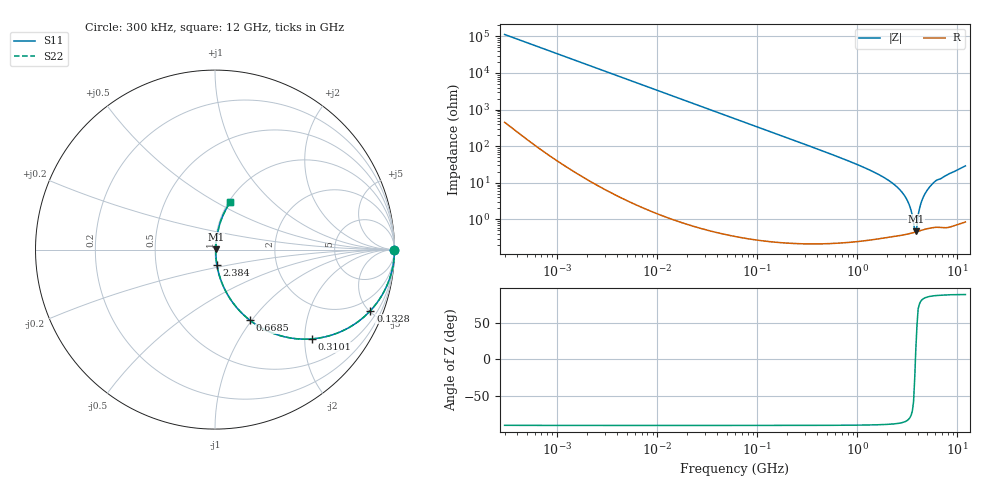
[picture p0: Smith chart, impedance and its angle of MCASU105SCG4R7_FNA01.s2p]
! MCASU105SCG4R7_FNA01  S-PARAMETER MODEL  ( Standard Model )
! Model Generated by TAIYO YUDEN Corporation (http://www.ty-top.com)
! Version 1.0
! TAIYO YUDEN Control No. 230609
! Copyright(c) 2023 TAIYO YUDEN CO.,LTD. All Rights Reserved.
! Product Description (link to TY-COMPAS)
! https://ds.yuden.co.jp/TYCOMPAS/or/detail?pn=MCASU105SCG4R7CFNA01&u=M
! Products Name : Multilayer Ceramic Capacitors
! Characteristics :
!  Capacitance : 4.7 [pF] , Rated Voltage : 50 [V] , TCC : CG / C0G
!  Case Size : 1.0 x 0.5 / 0.039 x 0.02 [mm/inch] , Thickness : 0.5 / 0.02 [mm/inch]
!  (Conditions: Temperature = 25 [degC] , DC Bias Voltage = 0 [V])
! External Node Assignments :
!  1  o---| |---o  2
! GND o---------o GND
! Frequency Range : 0.3MHz  -  12000MHz  [ 401 STEP ]
# MHZ S RI R 50
! Freq[MHz].  S11 Real  S11 Imag  S21 Real  S21 Imag  S12 Real  S12 Imag  S22 Real  S22 Imag
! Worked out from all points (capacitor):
!   401 points, 300 kHz to 12 GHz, reference 50 ohm
!   read as one part in series: C = 4.7 pF near 316.3 kHz
!   lowest |Z| = 471 mohm at 3.841 GHz (marker M1)
!   series resonance near 3.805 GHz, so ESL is about 370 pH
!   S11 on the Smith chart (normalised r, x): 300 kHz: open; 132.8 MHz: 1.00, -5.09; 310.1 MHz: 1.00, -2.17; 668.5 MHz: 1.00, -0.98; 2.384 GHz: 1.01, -0.17; 12 GHz: 1.02, +0.58
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0.3  1 -0.000886  4.32e-06 0.000886  4.32e-06 0.000886  1 -0.000886
1.769972  1 -0.00523  3.14e-05 0.00523  3.14e-05 0.00523  1 -0.00523
10.44266  0.999 -0.0308  0.000963 0.0308  0.000963 0.0308  0.999 -0.0308
60  0.9694 -0.1718  0.0306 0.1718  0.0306 0.1718  0.9694 -0.1718
132.8329  0.8661 -0.34  0.1339 0.34  0.1339 0.34  0.8661 -0.34
310.0777  0.5405 -0.4974  0.4595 0.4974  0.4595 0.4974  0.5405 -0.4974
353.9943  0.4735 -0.4982  0.5265 0.4982  0.5265 0.4982  0.4735 -0.4982
668.5285  0.1952 -0.3941  0.8048 0.3941  0.8048 0.3941  0.1952 -0.3941
1296.429  0.0528 -0.2178  0.9472 0.2178  0.9472 0.2178  0.0528 -0.2178
2088.533  0.0157 -0.1107  0.9843 0.1107  0.9843 0.1107  0.0157 -0.1107
2384.334  0.0107 -0.0845  0.9893 0.0845  0.9893 0.0845  0.0107 -0.0845
3107.553  0.00517 -0.0353  0.9948 0.0353  0.9948 0.0353  0.00517 -0.0353
3364.605  0.00456 -0.021  0.9954 0.021  0.9954 0.021  0.00456 -0.021
3642.919  0.0044 -0.00686  0.9956 0.00686  0.9956 0.00686  0.0044 -0.00686
3740.715  0.00445 -0.00215  0.9956 0.00215  0.9956 0.00215  0.00445 -0.00215
3841.137  0.00453 0.00121  0.9955 -0.00121  0.9955 -0.00121  0.00453 0.00121
3944.255  0.00465 0.00493  0.9953 -0.00493  0.9953 -0.00493  0.00465 0.00493
4270.516  0.00553 0.0242  0.9945 -0.0242  0.9945 -0.0242  0.00553 0.0242
4502.883  0.00652 0.0369  0.9935 -0.0369  0.9935 -0.0369  0.00652 0.0369
5278.635  0.0116 0.076  0.9884 -0.076  0.9884 -0.076  0.0116 0.076
6188.031  0.0195 0.1146  0.9805 -0.1146  0.9805 -0.1146  0.0195 0.1146
12000  0.0844 0.2637  0.9156 -0.2637  0.9156 -0.2637  0.0844 0.2637
